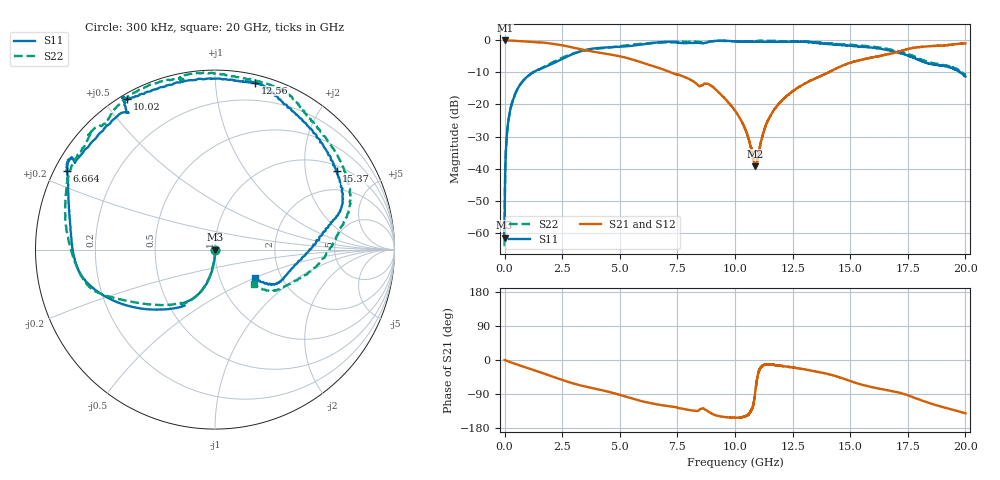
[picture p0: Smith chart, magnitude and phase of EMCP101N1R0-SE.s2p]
!EMCP101N1R0
!Johanson Technology Inc.
!www.johansontechnology.com
!Test Board Conditions:
!Substrate Type  RO4350B
!Substrate Thickness  10 mil
!Substrate Dk  3.66
!TL Type: GCPW
!TL Trace Width  20 mil
!TL Gap  10 mil
!PART MODE SINGLE ENDED (AKA BYPASS)
!DUT TOPOLOGY	SERIES-SHUNT
# MHz S  dB  R 50
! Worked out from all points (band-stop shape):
!   20001 points, 300 kHz to 20 GHz, reference 50 ohm
!   highest |S21| = 0.00 dB at 5.3 MHz (marker M1); lowest = -39.4 dB at 10.88 GHz (marker M2)
!   |S21| within 3 dB of the highest: start of sweep to 3.482 GHz; 17.35 GHz to end of sweep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
!   lowest |S11| = -61.5 dB at 1.3 MHz (marker M3), VSWR 1.00, Z = 50.1 - j0.0404 ohm
!   |S11| at or under -10 dB: start of sweep to 1.228 GHz; 1.228882 GHz to 1.229425 GHz (542.9 kHz wide, 0.0442 % of centre); 19.79 GHz to end of sweep
!   |S22| runs from -64.2 to -0.1 dB; largest |S21 - S12| = 0.018
!   S11 on the Smith chart (normalised r, x): 300 kHz: 1.00, +0.00; 6.664 GHz: 0.04, +0.25; 10.02 GHz: 0.02, +0.57; 12.56 GHz: 0.06, +1.27; 15.37 GHz: 1.19, +2.96; 20 GHz: 1.47, -0.50
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0.3  -56.57 18.9  -0.00 -0.2  0.00 -0.1  -64.24 55.5
1.3  -61.54 -28.8  -0.01 -0.0  -0.01 -0.1  -61.26 -32.8
5.3  -54.34 -69.0  -0.00 -0.1  -0.01 -0.1  -54.36 -68.3
105.298  -28.91 -91.2  -0.01 -2.4  -0.02 -2.4  -28.91 -91.7
158.298  -25.38 -93.1  -0.02 -3.6  -0.02 -3.6  -25.41 -93.6
545.292  -15.35 -101.9  -0.15 -12.0  -0.16 -12.0  -15.38 -102.6
2083.269  -7.23 -130.1  -1.02 -43.8  -1.02 -43.9  -6.83 -137.5
3334.25  -3.31 -159.0  -2.79 -67.6  -2.79 -67.7  -3.39 -158.4
6664.2  -0.59 151.9  -8.54 -117.5  -8.53 -117.5  -0.70 150.3
6667.2  -0.59 151.9  -8.55 -117.6  -8.54 -117.5  -0.70 150.3
8905.166  -0.40 121.8  -13.87 -138.7  -13.90 -138.9  -0.34 125.7
10000.15  -0.26 120.4  -21.91 -152.1  -21.89 -152.0  -0.27 101.3
10019.15  -0.28 120.2  -22.11 -152.1  -22.08 -151.6  -0.27 101.1
10466.14  -0.41 113.0  -28.12 -148.2  -28.07 -147.7  -0.31 101.0
10881.14  -0.43 102.1  -39.35 -84.1  -39.03 -85.2  -0.20 101.6
11516.13  -0.45 85.9  -23.82 -12.0  -23.94 -11.6  -0.11 94.5
12563.11  -0.39 76.6  -15.56 -20.1  -15.51 -20.2  -0.28 74.4
13334.1  -0.64 70.2  -12.35 -28.4  -12.33 -28.4  -0.48 62.5
15368.07  -1.88 32.8  -6.21 -62.6  -6.17 -62.2  -1.55 28.4
16667.05  -3.09 15.3  -4.24 -80.5  -4.34 -80.8  -2.72 11.8
18015.03  -6.26 -5.4  -2.07 -104.4  -2.08 -104.6  -5.79 -16.5
20000  -11.28 -35.7  -0.92 -140.7  -0.99 -140.2  -10.79 -42.3
